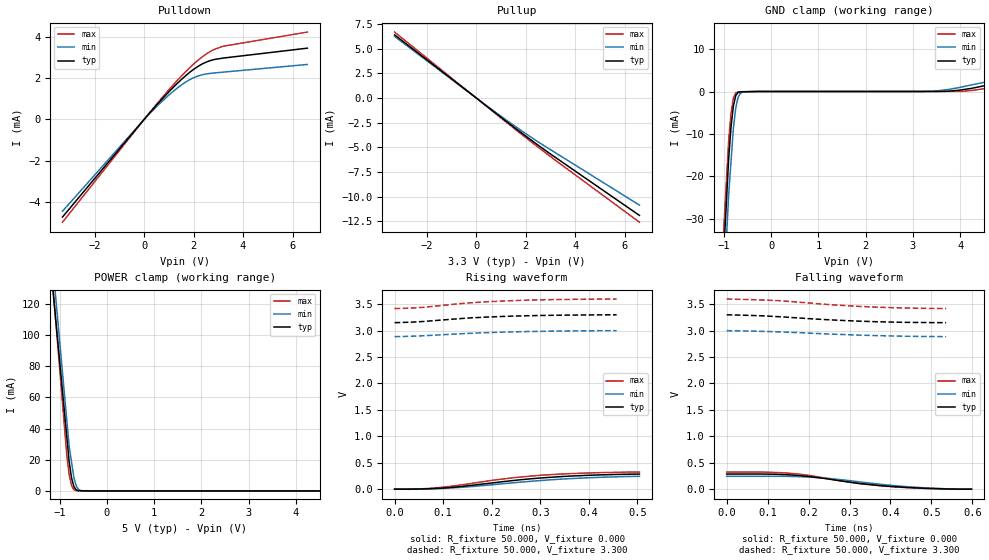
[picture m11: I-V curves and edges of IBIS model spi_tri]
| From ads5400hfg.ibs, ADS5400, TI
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[Model]   spi_tri
Model_type 3-state
Vref=0.000E+00
Rref=1.000E+06
Cref=0.000E+00
Vmeas=1.650E+00
C_comp   3.050E-13   2.910E-13   3.120E-13
[Voltage Range]   3.300E+00   3.000E+00   3.600E+00
[POWER Clamp Reference]   5.000E+00   4.750E+00   5.250E+00
[GND Clamp Reference]   0.000E+00   0.000E+00   0.000E+00
[Pullup Reference]   3.300E+00   3.000E+00   3.600E+00
[Pulldown Reference]   0.000E+00   0.000E+00   0.000E+00
[Temperature Range]   25   100   -40
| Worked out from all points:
|   slope of the pulldown table from 0 to 0.495 V, typ, clamps not added: 728 ohm
|   slope of the pullup table from 0 to 0.495 V, typ, clamps not added: 508 ohm
|   GND clamp passes 1 mA (typ) near -0.75 V on its own axis
|   POWER clamp passes 1 mA (typ) near -0.66 V on its own axis
|   rising waveform, R_fixture 50.000, V_fixture 0.000: 20-80 % time 184ps typ, 195ps min, 171ps max; typ from 0 V to 0.286 V
|   falling waveform, R_fixture 50.000, V_fixture 0.000: 20-80 % time 179ps typ, 177ps min, 172ps max; typ from 0.286 V to 0 V
|   rising waveform, R_fixture 50.000, V_fixture 3.300: 20-80 % time 158ps typ, 177ps min, 151ps max; typ from 3.15 V to 3.3 V
|   falling waveform, R_fixture 50.000, V_fixture 3.300: 20-80 % time 207ps typ, 223ps min, 200ps max; typ from 3.3 V to 3.15 V
[GND Clamp]
-5V       -891mA     -943.1mA   -837.3mA
-900mV    -16.02mA   -24.44mA   -11.71mA
-850mV    -8.487mA   -16.61mA   -5.236mA
-800mV    -3.473mA   -8.788mA   -1.618mA
-750mV    -981.8uA   -3.98mA    -351.4uA
-700mV    -229.6uA   -1.379mA   -87uA
-650mV    -69.04uA   -430.5uA   -74.72uA
-600mV    -59uA      -113.3uA   -62.45uA
3.2V      1.02uA     2.758uA    38.35uA
3.75V     58.88uA    475.6uA    44.46uA
4.3V      871.4uA    1.686mA    313.8uA
10V       13.86mA    14.97mA    13.35mA
[POWER Clamp]
-5V       1.364A     1.436A     1.557A
-1.1V     114.7mA    129.1mA    115.1mA
-1.05V    98.7mA     112.3mA    96.62mA
-850mV    34.64mA    45.28mA    22.71mA
-800mV    18.62mA    28.52mA    10.41mA
-750mV    8.359mA    18.51mA    3.385mA
-700mV    2.739mA    8.501mA    705.7uA
-650mV    661.8uA    3.183mA    173.9uA
-600mV    176.7uA    895.3uA    59.69uA
-550mV    85.04uA    199.8uA    52.67uA
-400mV    38.66uA    7.805uA    31.6uA
10V       0A         0A         0A
[Pullup]
-3.3V     6.391mA    6.233mA    6.673mA
500mV     -983.6uA   -937uA     -1.019mA
1.84V     -3.56mA    -3.343mA   -3.7mA
3.04V     -5.753mA   -5.302mA   -6.013mA
6.6V      -11.91mA   -10.87mA   -12.6mA
[Pulldown]
-3.3V     -4.715mA   -4.434mA   -4.966mA
160mV     225.6uA    203.7uA    239.7uA
600mV     821.3uA    732.7uA    876.6uA
1.3V      1.695mA    1.478mA    1.831mA
1.7V      2.133mA    1.82mA     2.33mA
1.98V     2.401mA    2.005mA    2.652mA
2.34V     2.676mA    2.155mA    3.014mA
2.54V     2.784mA    2.202mA    3.181mA
2.86V     2.901mA    2.248mA    3.396mA
3.2V      2.965mA    2.285mA    3.538mA
6.6V      3.443mA    2.656mA    4.22mA
[Rising Waveform]
R_fixture = 50.000
V_fixture = 0.000
V_fixture_min = 0.000
V_fixture_max = 0.000
|  time   V(typ)   V(min)   V(max)
0s        155.5uV    167.9uV    -130.6uV
54ps      2.954mV    2.104mV    6.783mV
91ps      15.93mV    11.29mV    29.45mV
140ps     52.97mV    36.58mV    84mV
208ps     124.8mV    89.61mV    175.8mV
248ps     166.5mV    122.9mV    219.5mV
304ps     213.2mV    165.4mV    265mV
391ps     259.2mV    211.9mV    303.7mV
468ps     280.3mV    236.2mV    320.8mV
504ps     285.6mV    243.3mV    322.8mV
[Falling Waveform]
R_fixture = 50.000
V_fixture = 0.000
V_fixture_min = 0.000
V_fixture_max = 0.000
|  time   V(typ)   V(min)   V(max)
0s        285.6mV    243.3mV    322.8mV
121ps     281.3mV    243.5mV    315.8mV
167ps     263.5mV    238.8mV    291.8mV
204ps     236.1mV    227.7mV    256.2mV
251ps     188.9mV    201.7mV    195.3mV
314ps     118.2mV    148mV      115.7mV
386ps     60.31mV    83.73mV    56.61mV
476ps     19.14mV    28.13mV    16.07mV
556ps     1.192mV    1.8mV      90.33uV
598ps     155.5uV    167.9uV    -130.6uV
[Rising Waveform]
R_fixture = 50.000
V_fixture = 3.300
V_fixture_min = 3.000
V_fixture_max = 3.600
|  time   V(typ)   V(min)   V(max)
0s        3.152V     2.887V     3.419V
24ps      3.158V     2.892V     3.424V
60ps      3.174V     2.904V     3.442V
119ps     3.217V     2.933V     3.498V
155ps     3.241V     2.949V     3.527V
189ps     3.257V     2.962V     3.546V
228ps     3.27V      2.973V     3.564V
275ps     3.283V     2.983V     3.578V
341ps     3.293V     2.993V     3.59V
457ps     3.3V       3V         3.598V
[Falling Waveform]
R_fixture = 50.000
V_fixture = 3.300
V_fixture_min = 3.000
V_fixture_max = 3.600
|  time   V(typ)   V(min)   V(max)
0s        3.3V       3V         3.598V
75ps      3.284V     2.989V     3.584V
123ps     3.266V     2.978V     3.569V
165ps     3.245V     2.966V     3.547V
194ps     3.23V      2.956V     3.528V
265ps     3.2V       2.932V     3.486V
314ps     3.183V     2.918V     3.463V
356ps     3.171V     2.908V     3.448V
441ps     3.157V     2.894V     3.428V
536ps     3.152V     2.887V     3.419V
[Ramp]
dV/dt_r   1.6701E-01/1.8302E-10   1.4147E-01/1.9428E-10   1.8896E-01/1.7150E-10
dV/dt_f   8.8777E-02/2.0512E-10   2.4000E+00/2.2325E-10   1.0776E-01/2.0125E-10
R_load = 50
